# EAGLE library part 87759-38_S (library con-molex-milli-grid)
HEADER
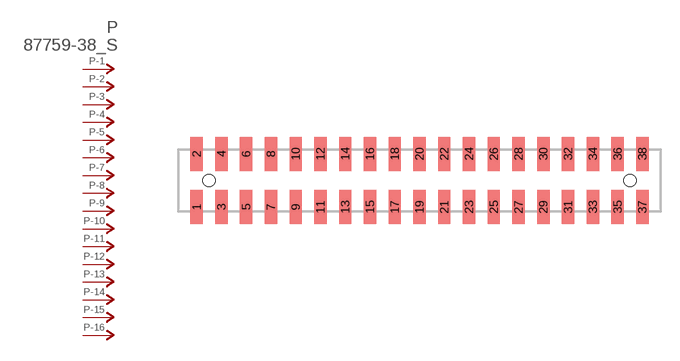
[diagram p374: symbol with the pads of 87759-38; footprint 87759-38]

Designator prefix P; gates -1=P-NV -2=P-N -3=P-N -4=P-N -5=P-N -6=P-N -7=P-N -8=P-N -9=P-N -10=P-N -11=P-N -12=P-N -13=P-N -14=P-N -15=P-N -16=P-N -17=P-N -18=P-N -19=P-N -20=P-N -21=P-N -22=P-N -23=P-N -24=P-N -25=P-N -26=P-N -27=P-N -28=P-N -29=P-N -30=P-N -31=P-N -32=P-N -33=P-N -34=P-N -35=P-N -36=P-N -37=P-N -38=P-N

## 87759-38_S  [87759-38]
1  -1:P  pas
2  -2:P  pas
3  -3:P  pas
4  -4:P  pas
5  -5:P  pas
6  -6:P  pas
7  -7:P  pas
8  -8:P  pas
9  -9:P  pas
10  -10:P  pas
11  -11:P  pas
12  -12:P  pas
13  -13:P  pas
14  -14:P  pas
15  -15:P  pas
16  -16:P  pas
17  -17:P  pas
18  -18:P  pas
19  -19:P  pas
20  -20:P  pas
21  -21:P  pas
22  -22:P  pas
23  -23:P  pas
24  -24:P  pas
25  -25:P  pas
26  -26:P  pas
27  -27:P  pas
28  -28:P  pas
29  -29:P  pas
30  -30:P  pas
31  -31:P  pas
32  -32:P  pas
33  -33:P  pas
34  -34:P  pas
35  -35:P  pas
36  -36:P  pas
37  -37:P  pas
38  -38:P  pas

## Footprint 87759-38 (pad centres in mm)
HEADER SMD Dual Row, Vertical
smd 1 x 2.75: 1 -18,-2.15; 2 -18,2.15; 3 -16,-2.15; 4 -16,2.15; 5 -14,-2.15; 6 -14,2.15; 7 -12,-2.15; 8 -12,2.15; 9 -10,-2.15; 10 -10,2.15; 11 -8,-2.15; 12 -8,2.15; 13 -6,-2.15; 14 -6,2.15; 15 -4,-2.15; 16 -4,2.15; 17 -2,-2.15; 18 -2,2.15; 19 0,-2.15; 20 0,2.15; 21 2,-2.15; 22 2,2.15; 23 4,-2.15; 24 4,2.15; 25 6,-2.15; 26 6,2.15; 27 8,-2.15; 28 8,2.15; 29 10,-2.15; 30 10,2.15; 31 12,-2.15; 32 12,2.15; 33 14,-2.15; 34 14,2.15; 35 16,-2.15; 36 16,2.15; 37 18,-2.15; 38 18,2.15
hole 1 at -17,0
hole 1 at 17,0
